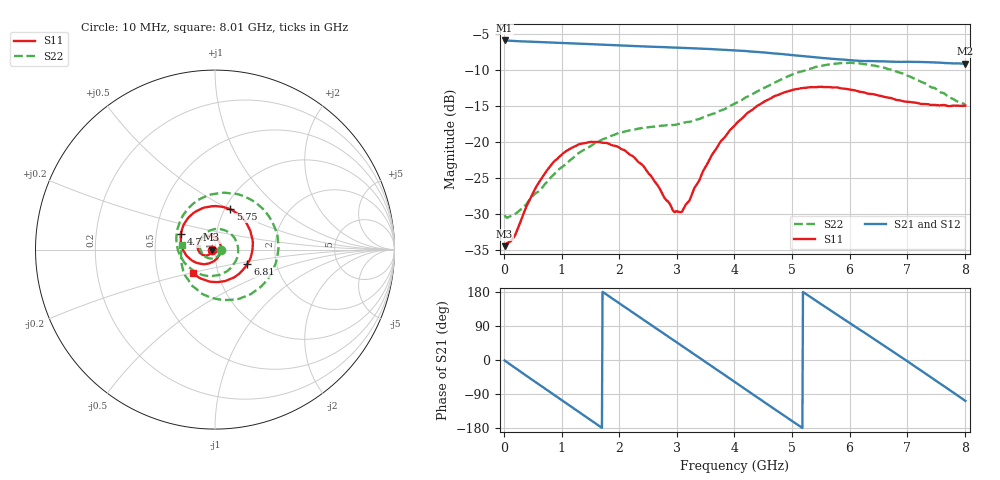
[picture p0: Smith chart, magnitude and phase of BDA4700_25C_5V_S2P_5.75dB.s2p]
!Agilent Technologies,E5071B,MY42404982,A.09.10
!Date: Mon Oct 20 13:28:48 2025
!Data & Calibration Information:
!Freq	S11:SOLT2(ON)	S21:SOLT2(ON)	S12:SOLT2(ON)	S22:SOLT2(ON)
# Hz S RI R 50
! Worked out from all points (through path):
!   801 points, 10 MHz to 8.01 GHz, reference 50 ohm
!   highest |S21| = -5.87 dB at 10 MHz (marker M1); lowest = -9.1 dB at 8.01 GHz (marker M2)
!   group delay of S21, straight-line fit = 286 ps
!   lowest |S11| = -34.4 dB at 10 MHz (marker M3), VSWR 1.04, Z = 48.1 - j0.106 ohm
!   |S11| at or under -10 dB: start of sweep to end of sweep
!   |S22| runs from -30.5 to -9.0 dB; largest |S21 - S12| = 0.0039
!   S11 on the Smith chart (normalised r, x): 10 MHz: 0.96, -0.00; 4.7 GHz: 0.67, +0.12; 5.75 GHz: 1.06, +0.51; 6.81 GHz: 1.42, -0.23; 8.01 GHz: 0.76, -0.20
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1e7  -0.019 -0.0011  0.5086 -0.0111  0.5087 -0.0114  0.0312 -0.00247
3.3e8  -0.0245 -0.0195  0.4085 -0.2901  0.4084 -0.2906  0.0227 -0.0268
7.1e8  -0.0511 -0.0329  0.1242 -0.4785  0.1237 -0.4788  -0.0137 -0.0494
1.02e9  -0.0806 -0.0215  -0.1508 -0.4647  -0.1512 -0.4648  -0.0575 -0.0363
1.35e9  -0.0973 0.0117  -0.383 -0.2933  -0.383 -0.2937  -0.0848 0.018
1.64e9  -0.0892 0.0467  -0.4733 -0.0598  -0.4736 -0.06  -0.0664 0.0767
1.93e9  -0.0614 0.0717  -0.4339 0.1838  -0.4343 0.1839  -0.00678 0.113
2.32e9  -0.0123 0.0727  -0.2086 0.4149  -0.2081 0.4152  0.0884 0.0871
2.68e9  0.0237 0.043  0.0837 0.451  0.0838 0.451  0.1293 -0.00313
3.08e9  0.0302 -0.0128  0.3561 0.2785  0.3548 0.2797  0.0835 -0.1062
3.53e9  -0.0154 -0.0691  0.4392 -0.0651  0.4396 -0.0661  -0.0427 -0.1465
4.01e9  -0.1117 -0.0697  0.2283 -0.3695  0.2285 -0.3694  -0.1729 -0.0689
4.35e9  -0.1728 -0.0112  -0.0266 -0.4236  -0.0271 -0.4247  -0.2148 0.0479
4.7e9  -0.1911 0.0859  -0.2661 -0.3161  -0.2655 -0.317  -0.1802 0.1872
5.02e9  -0.1487 0.1775  -0.3842 -0.1178  -0.3851 -0.1177  -0.0723 0.288
5.35e9  -0.0549 0.2349  -0.374 0.113  -0.3743 0.112  0.0913 0.3131
5.75e9  0.0848 0.2249  -0.2047 0.318  -0.2039 0.3181  0.2771 0.2151
6.19e9  0.1905 0.1182  0.0714 0.3598  0.0746 0.3602  0.3513 -0.0128
6.68e9  0.1996 -0.0417  0.3162 0.1777  0.3172 0.1775  0.2235 -0.2313
6.81e9  0.1804 -0.0787  0.3475 0.1012  0.3482 0.0992  0.1648 -0.2621
7.5e9  0.00856 -0.1808  0.2064 -0.2924  0.2056 -0.2928  -0.1374 -0.1898
8.01e9  -0.1237 -0.1301  -0.108 -0.3333  -0.108 -0.3338  -0.182 0.0275
